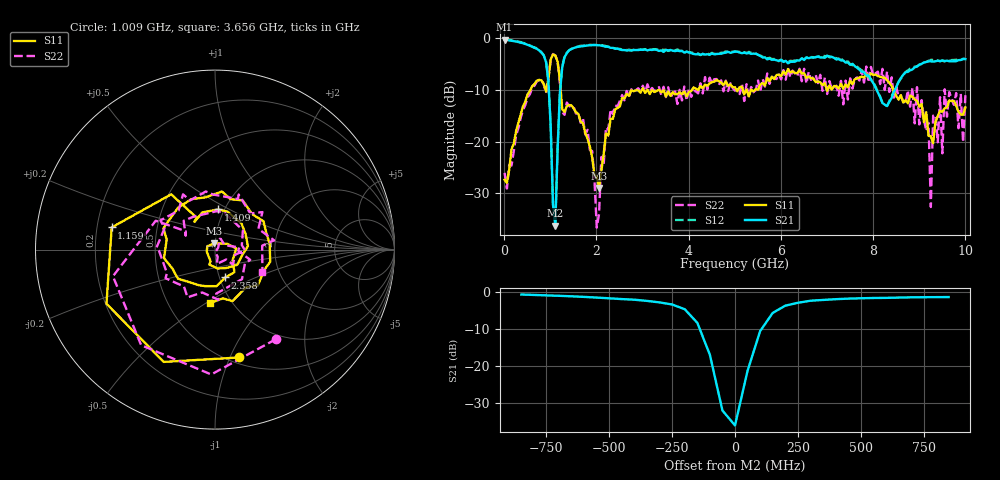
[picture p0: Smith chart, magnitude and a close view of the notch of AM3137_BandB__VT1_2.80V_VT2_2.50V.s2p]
! Date/Time: Tue, Nov 13, 2018 4:52 PM
! Network Analyzer: Agilent Technologies E8364B Rev: A.07.50.67
! Sweep from 0.010 to 10.000 GHz, 201 Points, Sweep Type: LIN
! Power Supply: 2.801 V, 0.001 A
# Hz S DB R 50
!freq MagS11 AngS11 MagS21 AngS21 MagS12 AngS12 MagS22 AngS22
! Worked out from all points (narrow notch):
!   201 points, 10 MHz to 10 GHz, reference 50 ohm
!   highest |S21| = -0.36 dB at 10 MHz (marker M1); lowest = -36.2 dB at 1.109 GHz (marker M2)
!   notch at M2: 32.9 dB deep, 148 MHz wide at half that depth
!   lowest |S11| = -28.9 dB at 2.058 GHz (marker M3), VSWR 1.07, Z = 49.5 + j3.53 ohm
!   |S11| at or under -10 dB: 1.225 GHz to 2.991 GHz (1.766 GHz wide, 83.8 % of centre); 3.022 GHz to 4.076 GHz (1.054 GHz wide, 29.7 % of centre); 8.433 GHz to end of sweep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
!   |S22| runs from -36.6 to -3.1 dB; largest |S21 - S12| = 0.034
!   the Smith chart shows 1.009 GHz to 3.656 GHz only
!   S11 on the Smith chart (normalised r, x): 1.009 GHz: 0.56, -1.08; 1.159 GHz: 0.26, +0.10; 1.409 GHz: 0.94, +0.44; 2.358 GHz: 1.07, -0.34; 3.656 GHz: 0.80, -0.52
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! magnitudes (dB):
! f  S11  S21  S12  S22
! 10 MHz  -27.4  -0.4  -0.3  -26.0
! 859.2 MHz  -8.9  -3.4  -3.4  -9.0
! 1.009 GHz  -4.2  -17.0  -17.0  -4.4
! 1.109 GHz  -3.4  -36.2  -36.2  -3.4
! 1.159 GHz  -4.6  -21.4  -21.3  -4.6
! 1.409 GHz  -13.0  -2.4  -2.4  -13.2
! 1.708 GHz  -16.5  -1.6  -1.5  -15.5
! 2.058 GHz  -28.9  -1.5  -1.4  -33.9
! 2.358 GHz  -15.6  -2.0  -1.9  -14.7
! 3.357 GHz  -10.0  -2.6  -2.3  -9.5
! 3.656 GHz  -10.5  -2.5  -2.5  -10.7
! 5.005 GHz  -9.6  -2.7  -2.6  -10.2
! 6.703 GHz  -7.8  -3.8  -3.8  -7.6
! 8.352 GHz  -8.7  -12.3  -12.2  -10.5
! 8.951 GHz  -12.1  -5.6  -5.5  -9.5
! 9.201 GHz  -18.9  -4.6  -4.4  -16.4
! 9.251 GHz  -19.0  -4.5  -4.3  -32.6
! 9.301 GHz  -20.3  -4.6  -4.3  -15.0
! 9.5 GHz  -14.3  -4.4  -4.4  -22.3
! 9.9 GHz  -14.8  -4.3  -4.3  -10.8
! 9.95 GHz  -14.9  -4.1  -4.1  -20.2
! 10 GHz  -13.4  -4.1  -4.0  -11.1
